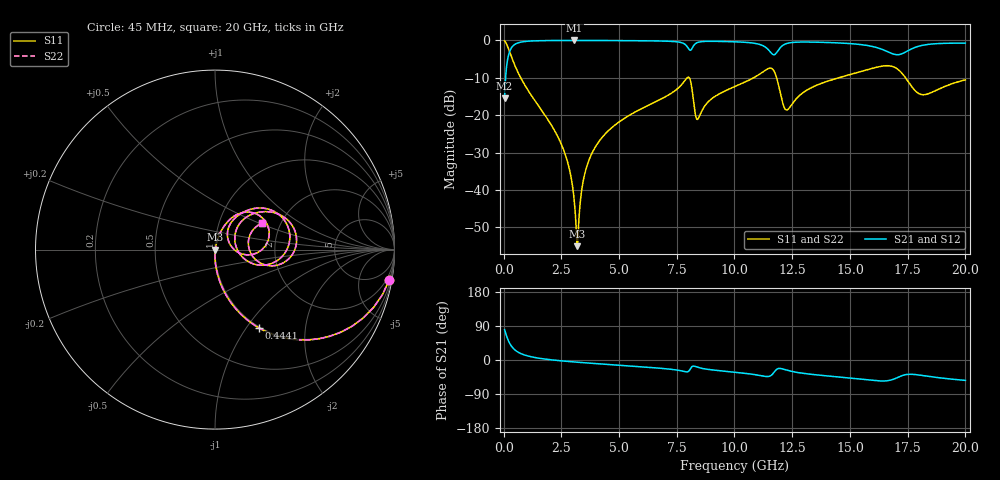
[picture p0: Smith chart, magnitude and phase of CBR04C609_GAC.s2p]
! S-parameter model data by Modelithics Inc.  support@modelithics.com 813-866-6335  Tampa FL USA
! S-Parameter data specifications:
! Substrate: 20-mil Rogers 4350B, substrate thickness, H=0.508mm, Dielectric constant, Er=3.75
! PCB Mounting Pad Footprint: Pad width, PadW=0.52mm , Pad length, PadL=0.52mm , Pad gap, PadG (edge-to-edge)=0.28mm , Reference planes=1.32mm apart
#  GHz  S  MA  R 50
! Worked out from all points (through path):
!   801 points, 45 MHz to 20 GHz, reference 50 ohm
!   highest |S21| = -0.02 dB at 3.063 GHz (marker M1); lowest = -15.4 dB at 45 MHz (marker M2)
!   group delay of S21, straight-line fit = 9.33 ps
!   lowest |S11| = -55.0 dB at 3.188 GHz (marker M3), VSWR 1.00, Z = 50.2 - j0.0391 ohm
!   |S11| at or under -10 dB: 743.4 MHz to 7.948 GHz (7.205 GHz wide, 166 % of centre); 8.043 GHz to 10.83 GHz (2.782 GHz wide, 29.5 % of centre); 11.82 GHz to 14.51 GHz (2.683 GHz wide, 20.4 % of centre)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
!   |S22| runs from -55.0 to -0.1 dB; largest |S21 - S12| = 0
!   S11 on the Smith chart (normalised r, x): 45 MHz: 1, -12; 444.1 MHz: 0.99, -1.15; 20 GHz: 1.60, +0.51
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0.045  0.9855 -9.8  0.1693 80.2  0.1693 80.2  0.9855 -9.8
0.219606  0.7646 -40.5  0.6441 49.5  0.6441 49.5  0.7646 -40.5
0.4441  0.5006 -60.7  0.865 29.2  0.865 29.2  0.5006 -60.7
0.992862  0.2321 -78.2  0.9717 11.6  0.9717 11.6  0.2321 -78.2
2.489488  0.04174 -90.0  0.9975 -2.2  0.9975 -2.2  0.04174 -90.0
2.863644  0.01824 -88.9  0.9981 -4.2  0.9981 -4.2  0.01824 -88.9
3.063194  0.007113 -81.1  0.9981 -5.2  0.9981 -5.2  0.007113 -81.1
3.187912  0.001779 -12.7  0.9981 -5.8  0.9981 -5.8  0.001779 -12.7
3.387462  0.01018 72.9  0.998 -6.8  0.998 -6.8  0.01018 72.9
3.711731  0.02573 77.4  0.9976 -8.3  0.9976 -8.3  0.02573 77.4
4.285437  0.05131 76.9  0.9964 -10.8  0.9964 -10.8  0.05131 76.9
6.704981  0.158 66.9  0.9824 -21.3  0.9824 -21.3  0.158 66.9
8.002056  0.3229 25.8  0.7823 -30.1  0.7823 -30.1  0.3229 25.8
8.4261  0.08985 34.2  0.9439 -19.5  0.9439 -19.5  0.08985 34.2
10.0225  0.2418 54.8  0.9577 -32.3  0.9577 -32.3  0.2418 54.8
11.59396  0.4239 10.5  0.6764 -40.4  0.6764 -40.4  0.4239 10.5
11.86834  0.2829 -17.9  0.7176 -23.1  0.7176 -23.1  0.2829 -17.9
12.26744  0.1176 15.3  0.9094 -26.9  0.9094 -26.9  0.1176 15.3
13.36496  0.2364 46.5  0.9489 -38.0  0.9489 -38.0  0.2364 46.5
16.68248  0.458 7.1  0.6948 -54.2  0.6948 -54.2  0.458 7.1
18.10428  0.1886 3.2  0.8548 -40.6  0.8548 -40.6  0.1886 3.2
20  0.2974 29.3  0.9192 -53.8  0.9192 -53.8  0.2974 29.3
